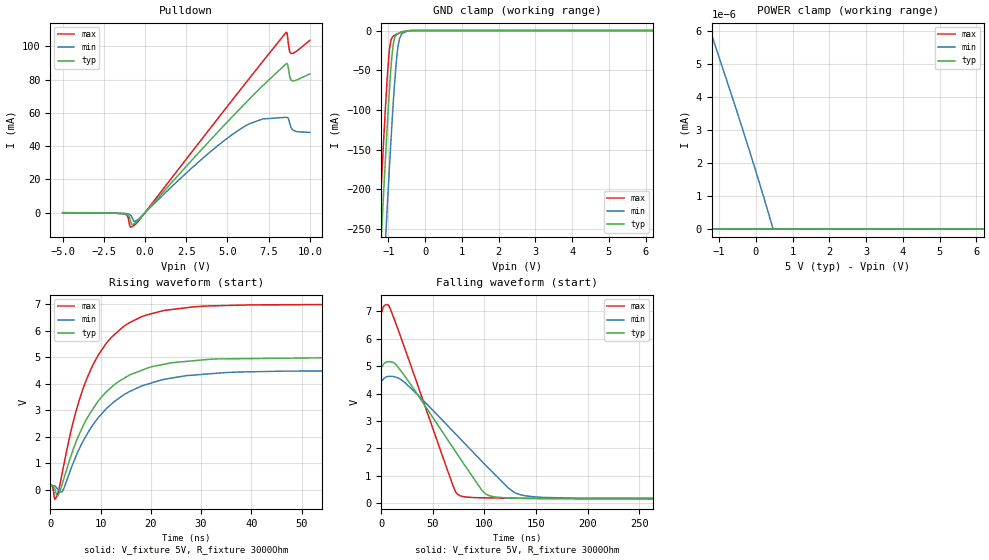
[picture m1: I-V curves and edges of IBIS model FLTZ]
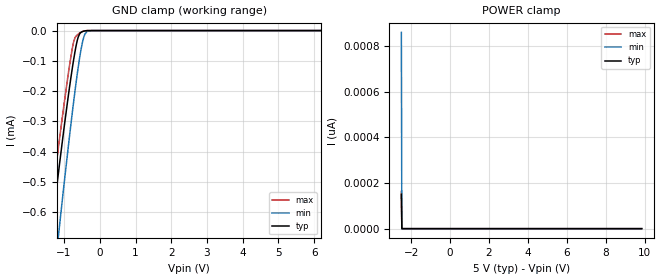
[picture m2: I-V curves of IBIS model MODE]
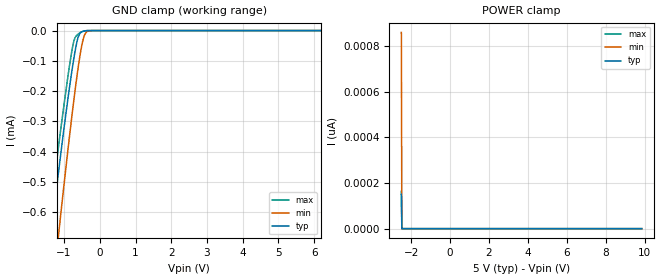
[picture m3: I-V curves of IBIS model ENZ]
| Texas Instruments Incorporated
| USB 2-Ch Data Line Short-to-Battery, Short-to-VBUS, and IEC ESD Protection
| Marketing part#   Voltage Range   Package-type   #pins/pkg drawing
| TPD2S703-Q1DSK   4.5V - 7.0V   QFP   10-pin DSK
| TPD2S703-Q1DGS   4.5V - 7.0V   VSSOP   10-pin DGS
[IBIS Ver]   4.1
[File name]   tpd2s703.ibs
[File Rev]   1.0
[Date]   01/11/2017
[Source]   Model built from spectre simulations at:
   Texas Instruments Incorporated.
   Webench Design Center
   12500 TI Blvd
   Dallas, TX -75243
   For Support e-mail: elab_ibis@list.ti.com
[Notes]   Revision History
   Rev 1.0: 01/11/2017
   - Non monotonic behavior result of circuit behavior
   - ccomp values are based on PVT settings:
   MIN: Low Voltage, High Temperature, Weak Process
   TYP: Nominal Voltage, Nominal Temperature, Nominal Process
   MAX: High Voltage, Low Temperature, Fast Process
   - C_comp although listed in numerical order of value are obtained from varying PVT conditions.
   For PVT conditions for each specific value, refer to the buffer description under respective [Model].
   IBIS model user is responsible for using appropriate C_comp to simulate for Signal Integrity.
[Disclaimer]  This model is designed as an aid for customers of Texas Instruments
 TI and its licensors and suppliers make no warranties, either expressed
 or implied, with respect to this  model, including the warranties of
 merchantability or fitness for a particular purpose.
 The model is provided solely on an "as is" basis. The entire risk as to
 its quality and performance is with the customer.
[Copyright] (C)Copyright 2017 Texas Instruments Incorporated.
   All rights reserved.
[Component]   TPD2S703DSK
[Manufacturer]  Texas Instruments Incorporated
[Package]   |10-pin QFN DSK package
|   typ   min   max
R_pkg   0.0661   0.0296   0.1020
L_pkg   1.0085n   0.6746n   1.4629n
C_pkg   0.1738p   0.1412p   0.2316p
[Pin]   signal_name   model_name   R_pin   L_pin   C_pin
1   VD-   NC   0.10196  1.46292n  0.17126p
2   VD+   NC   0.07733  1.09469n  0.16457p
3   GND   GND   0.02964  0.81904n  0.23155p
4   /FLT   FLTZ   0.06857  0.96927n  0.15381p
5   /EN   ENZ   0.07293  1.03692n  0.14118p
6   MODE   MODE   0.07120  1.00522n  0.14185p
7   VPWR   POWER   0.03440  0.67461n  0.18548p
8   VREF   NC   0.04024  0.69368n  0.22415p
9   D+   NC   0.08776  1.23840n  0.17661p
10   D-   NC   0.07714  1.08988n  0.14746p
[Component]   TPD2S703DGS
[Manufacturer]  Texas Instruments Incorporated
[Package]   |10-pin VSSOP DGS package
|   typ   min   max
R_pkg   0.0398   0.0206   0.0596
L_pkg   1.6054n   1.3021n   2.0762n
C_pkg   0.2903p   0.2438p   0.3575p
[Pin]   signal_name   model_name   R_pin   L_pin   C_pin
1   VD-   NC   0.05961  2.07621n  0.27834p
2   VD+   NC   0.04570  1.67647n  0.28692p
3   GND   GND   0.02061  1.45981n  0.35748p
4   /FLT   FLTZ   0.04034  1.53009n  0.27325p
5   /EN   ENZ   0.04295  1.61342n  0.24381p
6   MODE   MODE   0.04206  1.57806n  0.24569p
7   VPWR   POWER   0.02290  1.30205n  0.30877p
8   VREF   NC   0.02606  1.30223n  0.35443p
9   D+   NC   0.05183  1.83296n  0.30131p
10   D-   NC   0.04589  1.68223n  0.25296p
| Models and submodels in the file (3): FLTZ (Open_sink), MODE (Input), ENZ (Input)
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|   Model FLTZ
[Model]   FLTZ
Model_type   Open_sink
Polarity   Non-Inverting
Vmeas = 2.5
Vref = 5
Cref = 1pF
Rref = 3000
|   typ   min   max
|   (nom PVT)   (slow PVT)   (fast PVT)
C_comp   0.028p   0.016p   0.035p
|C_comp (ON state)   0.028p   0.016p   0.035p
|C_comp (OFF state)   0.113p   0.055p   0.186p
| Where   nom PVT is  Nominal Process, 5V, 27C
|   Fast PVT is Strong Process, 7V, -40C
|   Slow PVT is Weak Process, 4.5V, 125C
[Voltage Range]   5   4.5   7
[Temperature Range]   27   125   -40
[Pullup Reference]   5   4.5   7
[Pulldown Reference]   0   0   0
[Power Clamp Reference]   5   4.5   7
[GND Clamp Reference]   0   0   0
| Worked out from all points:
|   slope of the pulldown table from 0 to 0.75 V, typ, clamps not added: 89 ohm
|   GND clamp passes 1 mA (typ) near -0.55 V on its own axis
|   POWER clamp passes 1 mA (typ) near -3.61 V on its own axis
|   falling waveform, V_fixture 5V, R_fixture 3000Ohm: 20-80 % time 51.7ns typ, 66.9ns min, 38ns max; typ from 5 V to 0.142 V
|   rising waveform, V_fixture 5V, R_fixture 3000Ohm: 20-80 % time 9.32ns typ, 10.4ns min, 8.24ns max; typ from 0.142 V to 5 V
[Pulldown]
|   Voltage   I(typ)   I(min)   I(max)
-5V       -54.36uA   -50.06uA   -52.17uA
-1.25V    -655.2uA   -465.2uA   -794.3uA
-1.055V   -1.372mA   -767.3uA   -2.353mA
-890mV    -4.741mA   -1.532mA   -8.727mA
-665mV    -6.676mA   -5.23mA    -7.632mA
3.79V     41.81mA    35.14mA    48.65mA
6.28V     67.81mA    53.24mA    80.16mA
8.56V     89.57mA    57.34mA    108.4mA
8.65V     89mA       57.1mA     105.5mA
8.755V    82.94mA    54.62mA    97.57mA
8.86V     79.82mA    51.17mA    95.77mA
10V       83.48mA    48.26mA    103.6mA
[GND Clamp]
|   Voltage   I(typ)   I(min)   I(max)
-5V       -3.997A    -4.091A    -3.941A
-1.25V    -313.9mA   -420mA     -247.4mA
-1.16V    -232mA     -337.6mA   -165.9mA
-1.07V    -153.2mA   -257.1mA   -89.57mA
-1.01V    -103.9mA   -205.1mA   -45.73mA
-965mV    -70.1mA    -167.3mA   -22.06mA
-875mV    -20.18mA   -96.93mA   -7.627mA
-815mV    -7.834mA   -56.7mA    -5.597mA
-755mV    -4.578mA   -26.43mA   -4.125mA
-695mV    -3.099mA   -10.04mA   -2.894mA
-635mV    -2.033mA   -4.182mA   -1.826mA
10V       0A         0A         0A
[POWER Clamp]
|   Voltage   I(typ)   I(min)   I(max)
-5V       205.3mA    109.3mA    546.4mA
-3.53V    20.22uA    15.88nA    303.4mA
-2.705V   0A         11.5nA     167.9mA
-1.55V    0A         7.076nA    103.9uA
-1.25V    0A         6.048nA    0A
-785mV    0A         4.489nA    0A
-380mV    0A         3.102nA    0A
85mV      0A         1.447nA    0A
460mV     0A         28.44pA    0A
490mV     0A         0A         0A
10V       0A         0A         0A
[Ramp]
R_load = 3000
|   typ   min   max
dV/dt_r   2.91473/9.32214e-09   2.61235/1.04356e-08   4.09571/8.24554e-09
dV/dt_f   2.9145/5.15992e-08   2.61148/6.67289e-08   4.09567/3.80061e-08
[Falling Waveform]
V_fixture = 5V
V_fixture_min = 4.5V
V_fixture_max = 7V
R_fixture = 3000Ohm
C_fixture = 0F
|   Time   V(typ)   V(min)   V(max)
0s        5V         4.5V       7V
4.7ns     5.147V     4.603V     7.25V
8.626ns   5.168V     4.633V     7.125V
23.93ns   4.593V     4.371V     5.554V
69.64ns   2.027V     2.629V     651.2mV
76.66ns   1.63V      2.353V     271.3mV
101.7ns   331.1mV    1.373V     197.7mV
128.3ns   181.1mV    413mV      184.2mV
141.4ns   172.6mV    263mV      183.9mV
499.9ns   142.5mV    147.5mV    173.9mV
[Rising Waveform]
V_fixture = 5V
V_fixture_min = 4.5V
V_fixture_max = 7V
R_fixture = 3000Ohm
C_fixture = 0F
|   Time   V(typ)   V(min)   V(max)
0s        142.1mV    146mV      173.8mV
885.3ps   28.43mV    138.9mV    -359.1mV
1.325ns   -237.1mV   61.56mV    -232.3mV
2.371ns   215.5mV    -72.27mV   627.9mV
5.887ns   2.146V     1.593V     3.462V
8.316ns   3V         2.405V     4.65V
11.11ns   3.691V     3.053V     5.525V
18.16ns   4.511V     3.92V      6.536V
28.55ns   4.875V     4.333V     6.912V
499.9ns   5V         4.5V       7V
|   Model MODE
[Model]   MODE
Model_type   Input
Vinl = .8
Vinh = 1.2
|   typ   min   max
|   (nom PVT)   (fast PVT)   (slow PVT)
C_comp   0.373p   0.333p   0.380p
| Where   nom PVT is  Nominal Process, 5V, 27C
|   Fast PVT is Strong Process, 7V, -40C
|   Slow PVT is Weak Process, 4.5V, 125C
[Voltage Range]   5   4.5   7
[Temperature Range]   27   125   -40
[Power Clamp Reference]   5   4.5   7
[GND Clamp Reference]   0   0   0
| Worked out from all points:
|   GND clamp passes 1 mA (typ) near -1.68 V on its own axis
[GND Clamp]
|   Voltage   I(typ)   I(min)   I(max)
-2.5V     -1.888mA   -2.297mA   -1.775mA
-1.45V    -762uA     -1.009mA   -667.6uA
-1.35V    -661uA     -894.9uA   -568.7uA
-1.188V   -500.2uA   -712.5uA   -413.7uA
-1.1V     -415.8uA   -616.3uA   -333.4uA
-875mV    -211.1uA   -377.7uA   -138uA
-750mV    -110.1uA   -253uA     -47.68uA
-625mV    -30.3uA    -139uA     -13.64uA
-487.5mV  -3.407uA   -40.3uA    -3.146uA
-412.5mV  -937.2nA   -11.02uA   -701.1nA
-237.5mV  0A         -27.79nA   0A
9.838V    0A         0A         0A
[POWER Clamp]
|   Voltage   I(typ)   I(min)   I(max)
-2.5V     151.1pA    860.6pA    163.4pA
-2.475V   0A         0A         0A
-2.462V   0A         0A         0A
9.838V    0A         0A         0A
|   Model ENZ
[Model]   ENZ
Model_type   Input
Vinl = .8
Vinh = 1.2
|   typ   min   max
|   (nom PVT)   (fast PVT)   (slow PVT)
C_comp   0.373p   0.333p   0.380p
| Where   nom PVT is  Nominal Process, 5V, 27C
|   Fast PVT is Strong Process, 7V, -40C
|   Slow PVT is Weak Process, 4.5V, 125C
[Voltage Range]   5   4.5   7
[Temperature Range]   27   125   -40
[Power Clamp Reference]   5   4.5   7
[GND Clamp Reference]   0   0   0
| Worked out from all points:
|   GND clamp passes 1 mA (typ) near -1.68 V on its own axis
[GND Clamp]
|   Voltage   I(typ)   I(min)   I(max)
-2.5V     -1.888mA   -2.297mA   -1.775mA
-1.45V    -762uA     -1.009mA   -667.6uA
-1.35V    -661uA     -894.9uA   -568.7uA
-1.188V   -500.2uA   -712.5uA   -413.7uA
-1.1V     -415.8uA   -616.3uA   -333.4uA
-875mV    -211.1uA   -377.7uA   -138uA
-750mV    -110.1uA   -253uA     -47.68uA
-625mV    -30.3uA    -139uA     -13.64uA
-487.5mV  -3.407uA   -40.3uA    -3.146uA
-412.5mV  -937.2nA   -11.02uA   -701.1nA
-237.5mV  0A         -27.8nA    0A
9.838V    0A         0A         0A
[POWER Clamp]
|   Voltage   I(typ)   I(min)   I(max)
-2.5V     151.1pA    860.6pA    163.4pA
-2.475V   0A         0A         0A
-2.462V   0A         0A         0A
9.838V    0A         0A         0A
